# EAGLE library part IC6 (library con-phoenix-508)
PHOENIX
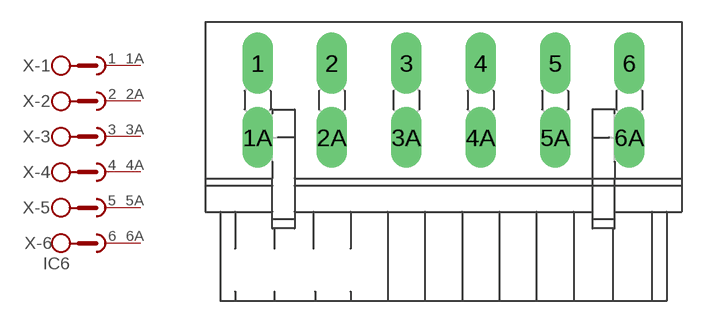
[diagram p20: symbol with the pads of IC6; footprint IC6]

Designator prefix X; gates -1=SKB2 -2=SKB2 -3=SKB2 -4=SKB2 -5=SKB2 -6=SKB2V

## IC6 (OC_FARNELL: unknown; OC_NEWARK: unknown)  [IC6]
1  -1:1  pas
1A  -1:2  pas
2  -2:1  pas
2A  -2:2  pas
3  -3:1  pas
3A  -3:2  pas
4  -4:1  pas
4A  -4:2  pas
5  -5:1  pas
5A  -5:2  pas
6  -6:1  pas
6A  -6:2  pas

## Footprint IC6 (pad centres in mm)
PHOENIX
drill 1.397 long: 1 -12.7,2.54; 1A -12.7,-2.54; 2 -7.62,2.54; 2A -7.62,-2.54; 3 -2.54,2.54; 3A -2.54,-2.54; 4 2.54,2.54; 4A 2.54,-2.54; 5 7.62,2.54; 5A 7.62,-2.54; 6 12.7,2.54; 6A 12.7,-2.54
